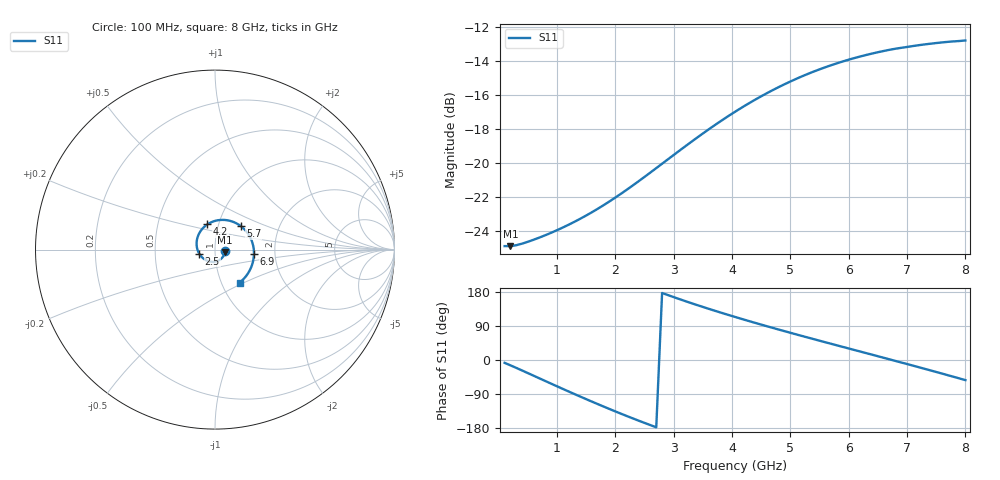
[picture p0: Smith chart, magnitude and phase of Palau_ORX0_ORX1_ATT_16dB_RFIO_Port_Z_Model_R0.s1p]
! Created Wed Sep 30 08:54:42 2020
! Palau ORX0/ORX1 RFIO Port Impedance Model.
! Attenuation : 16 dB.
! Revision		: R0.
! Impedance Mode 	: Balanced Differential-Mode.
! Impedance Format 	: Series Equivalent Differential Impedance (SEDZ).
# hz S ma R 100
! 1 Port Network Data from SP1.SP block
! freq  magS11  angS11
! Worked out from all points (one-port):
!   80 points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, 100 MHz to 8 GHz, reference 100 ohm
!   lowest |S11| = -24.9 dB at 200 MHz (marker M1), VSWR 1.12, Z = 112 - j3.1 ohm
!   |S11| at or under -10 dB: start of sweep to end of sweep
!   S11 on the Smith chart (normalised r, x): 100 MHz: 1.12, -0.02; 2.5 GHz: 0.84, -0.04; 4.2 GHz: 0.88, +0.25; 5.7 GHz: 1.28, +0.35; 6.9 GHz: 1.55, -0.08; 8 GHz: 1.22, -0.47
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1e8  0.0569 -7.5
2e8  0.05688 -14.1
6e8  0.05944 -41.6
1.1e9  0.06458 -76.4
1.4e9  0.06855 -96.7
1.6e9  0.07166 -110.0
1.8e9  0.07517 -123.0
2.1e9  0.08128 -142.0
2.5e9  0.09104 -166.1
2.8e9  0.09951 176.8
3.1e9  0.1088 160.5
3.3e9  0.1154 150.1
3.6e9  0.1257 135.1
3.8e9  0.1327 125.4
4.1e9  0.1433 111.3
4.2e9  0.1468 106.8
4.5e9  0.1573 93.4
4.7e9  0.1641 84.6
5.1e9  0.177 67.6
5.4e9  0.186 55.1
5.7e9  0.1942 42.7
6.1e9  0.2039 26.3
6.5e9  0.212 9.9
6.9e9  0.2184 -6.6
7.1e9  0.2211 -14.8
7.5e9  0.2256 -31.6
7.7e9  0.2275 -40.1
8e9  0.2296 -53.1
